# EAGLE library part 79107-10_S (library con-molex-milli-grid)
RECEPTACAL
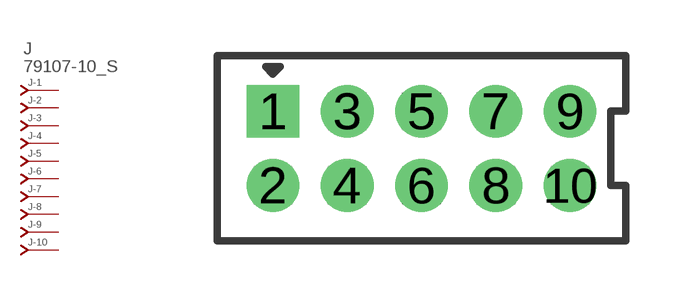
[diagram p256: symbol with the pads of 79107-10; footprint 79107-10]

Designator prefix J; gates -1=J-NV -2=J-N -3=J-N -4=J-N -5=J-N -6=J-N -7=J-N -8=J-N -9=J-N -10=J-N

## 79107-10_S  [79107-10]
1  -1:J  pas
2  -2:J  pas
3  -3:J  pas
4  -4:J  pas
5  -5:J  pas
6  -6:J  pas
7  -7:J  pas
8  -8:J  pas
9  -9:J  pas
10  -10:J  pas

## Footprint 79107-10 (pad centres in mm)
RECEPTACAL Dual Row, Vertical, Through-Hole
drill 0.914 square: 1 -4,1
drill 0.914: 2 -4,-1; 3 -2,1; 4 -2,-1; 5 0,1; 6 0,-1; 7 2,1; 8 2,-1; 9 4,1; 10 4,-1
